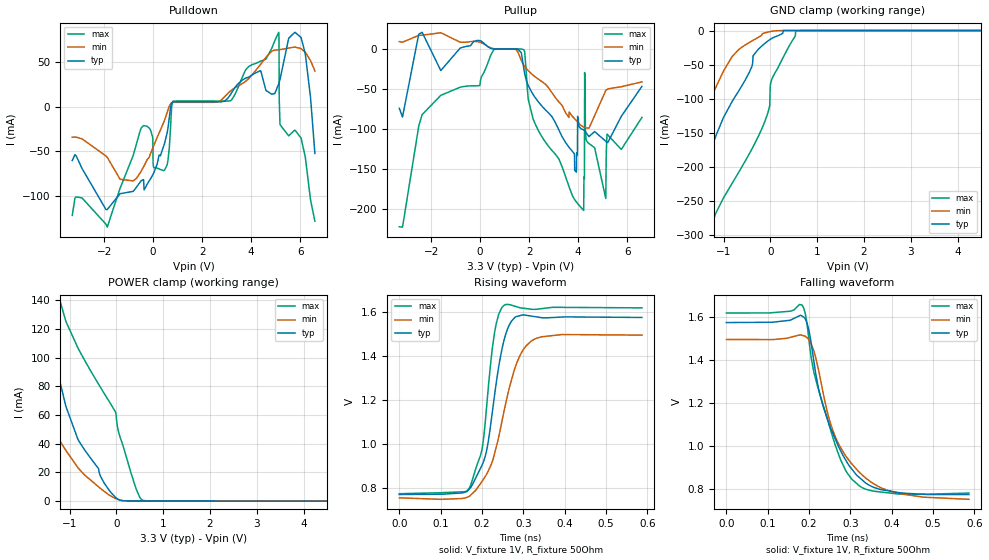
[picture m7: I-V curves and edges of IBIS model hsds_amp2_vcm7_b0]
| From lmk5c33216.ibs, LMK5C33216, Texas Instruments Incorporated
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[Model]   hsds_amp2_vcm7_b0
Model_type   Output
Polarity   Non-Inverting
Vmeas = 1.2
Vref = 1
Cref = 0pF
Rref = 50
|   typ   min   max
C_comp   0.65pF   0.575pF   0.725pF
[Voltage Range]   3.3   3.135   3.465
[Temperature Range]   50   135   -40
[Pullup Reference]   3.3   3.135   3.465
[Pulldown Reference]   -0   0   -0
[Power Clamp Reference]   3.3   3.135   3.465
[GND Clamp Reference]   0   0   0
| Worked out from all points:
|   slope of the pulldown table from 0 to 0.495 V, typ, clamps not added: 13.1 ohm
|   slope of the pullup table from 0 to 0.495 V, typ, clamps not added: 49.4 ohm
|   falling waveform, V_fixture 1V, R_fixture 50Ohm: 20-80 % time 78.7ps typ, 87.3ps min, 71.6ps max; typ from 1.58 V to 0.772 V
|   rising waveform, V_fixture 1V, R_fixture 50Ohm: 20-80 % time 40.8ps typ, 58.5ps min, 30.7ps max; typ from 0.771 V to 1.58 V
[Pulldown]
|   Voltage   I(typ)   I(min)   I(max)
-3.3V     -60.58mA   -34.5mA    -122.3mA
-1.874V   -115.7mA   -56.96mA   -135.5mA
-815.1mV  -95.3mA    -83.55mA   -55.05mA
-250.8mV  -87.64mA   -60.02mA   -22.2mA
462mV     -41.66mA   -15.43mA   -71.47mA
778.8mV   4.599mA    4.4mA      4.218mA
3.165V    13.91mA    17.71mA    6.774mA
5.125V    25.53mA    63.8mA     83.35mA
5.145V    27.36mA    63.85mA    8.329mA
5.184V    31.46mA    63.98mA    -20.67mA
6.036V    77.6mA     65.09mA    -35.45mA
6.6V      -52.72mA   40.01mA    -128.7mA
[GND Clamp]
|   Voltage   I(typ)   I(min)   I(max)
-3.3V     -892.9mA   -765.6mA   -1.068A
-1.924V   -314.6mA   -288.5mA   -459.9mA
-1.815V   -287mA     -251.4mA   -425.6mA
-1.478V   -218.2mA   -143.5mA   -333.1mA
-1.162V   -154.3mA   -82.94mA   -268mA
-815.1mV  -104mA     -38.12mA   -224.4mA
-171.6mV  -22.09mA   -4.573mA   -142.5mA
-13.2mV   -13.46mA   -1.685mA   -109.6mA
-3.3mV    -13.01mA   -1.546mA   -81.32mA
26.4mV    -11.77mA   -1.169mA   -72.35mA
551.1mV   0A         -83.65nA   -742uA
6.6V      0A         0A         0A
[Pullup]
|   Voltage   I(typ)   I(min)   I(max)
-3.3V     -74.05mA   9.29mA     -222.2mA
-2.369V   20.88mA    17.26mA    -82.04mA
570.9mV   24.97uA    290.1uA    -435.7uA
1.789V    -26.15mA   -20.58mA   -1.241mA
3.858V    -152mA     -87.31mA   -188.3mA
4.224V    -101mA     -97.5mA    -201.7mA
4.254V    -101.7mA   -97.86mA   -161.9mA
4.264V    -102mA     -97.97mA   -29.46mA
4.323V    -104.6mA   -98.58mA   -113mA
5.125V    -115.3mA   -51.81mA   -186.8mA
5.174V    -116.8mA   -50.63mA   -106.8mA
6.6V      -46.62mA   -41.07mA   -85.43mA
[POWER Clamp]
|   Voltage   I(typ)   I(min)   I(max)
-3.3V     330.7mA    180mA      566.4mA
-2.736V   200mA      135.8mA    401.6mA
-1.647V   138.3mA    65.17mA    197.7mA
-1.459V   117.6mA    55.06mA    168.7mA
-1.082V   66.76mA    35.64mA    126mA
-815.1mV  42.67mA    23.06mA    106.5mA
-3.3mV    2.23mA     1.644mA    59.85mA
46.2mV    1.16mA     1.045mA    48.48mA
313.5mV   86.42uA    94.45uA    19.62mA
491.7mV   74.41uA    72.76uA    3.272mA
570.9mV   69.96uA    68.47uA    464.4uA
6.6V      0A         0A         0A
[Ramp]
R_load = 50
|   typ   min   max
dV/dt_r   0.482846/4.05917e-11   0.443795/5.83946e-11   0.50691/3.0555e-11
dV/dt_f   0.482044/7.84886e-11   0.44798/8.68343e-11   0.504814/7.14129e-11
[Falling Waveform]
V_fixture = 1V
V_fixture_min = 0.95V
V_fixture_max = 1.05V
R_fixture = 50Ohm
C_fixture = 0F
|   Time   V(typ)   V(min)   V(max)
0s        1.576V     1.496V     1.62V
182.8ps   1.606V     1.516V     1.658V
198.8ps   1.547V     1.497V     1.511V
211.1ps   1.403V     1.446V     1.35V
224.7ps   1.252V     1.338V     1.251V
259.4ps   1.05V      1.063V     1.027V
288.2ps   935mV      954.4mV    886.3mV
322ps     851.4mV    875.9mV    812.3mV
411.7ps   783mV      779.8mV    775.6mV
586.8ps   772.2mV    749.8mV    778.9mV
[Rising Waveform]
V_fixture = 1V
V_fixture_min = 0.95V
V_fixture_max = 1.05V
R_fixture = 50Ohm
C_fixture = 0F
|   Time   V(typ)   V(min)   V(max)
0s        771.1mV    755.9mV    774.6mV
169ps     795.5mV    762.5mV    799.1mV
200ps     904mV      830.2mV    976.4mV
208.7ps   950.9mV    855.5mV    1.117V
221.8ps   1.1V       905.1mV    1.383V
230.8ps   1.229V     960.3mV    1.511V
253.7ps   1.475V     1.153V     1.632V
285.7ps   1.581V     1.376V     1.623V
325.1ps   1.58V      1.476V     1.613V
586.8ps   1.576V     1.496V     1.619V
